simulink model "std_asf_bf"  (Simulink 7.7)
settings: Solver=ode45  StartTime=0.0  StopTime=10.0  RelTol=1e-3
libraries: cstblocks x1

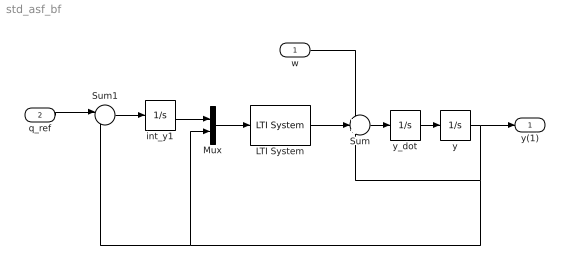
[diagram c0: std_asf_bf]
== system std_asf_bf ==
  w : Inport
  q_ref : Inport  Port=2
  LTI System : cstblocks/LTI System  SystemSampleTime=-1  sys=K_struct  IC=[]
  Mux : Mux  Inputs=2
  Sum : Sum  Inputs=+++
  Sum1 : Sum  Inputs=|-+
  int_y1 : Integrator
  y : Integrator
  y_dot : Integrator  InitialCondition=-1
  y(1) : Outport
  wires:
  Sum/1 -> y_dot/1
  y_dot/1 -> y/1
  y/1 -> y(1)/1, Sum1/2, Mux/2, Sum/3
  q_ref/1 -> Sum1/1
  Sum1/1 -> int_y1/1
  Mux/1 -> LTI System/1
  int_y1/1 -> Mux/1
  LTI System/1 -> Sum/2
  w/1 -> Sum/1
